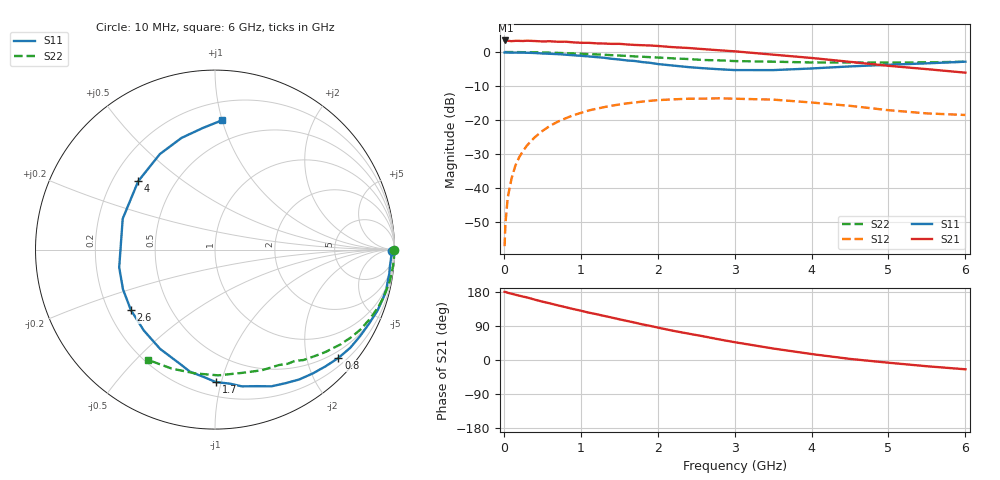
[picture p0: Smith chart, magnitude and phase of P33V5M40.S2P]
! SIEMENS Small Signal Semiconductors
! BFP181
! Si NPN RF Bipolar Junction Transistor in SOT143
! VCE = 3.5 V  IC = 0.4 mA
! Common Emitter S-Parameters:  March  1996
# GHz  S  MA  R  50
!  f  S11  S21  S12  S22
! GHz  MAG  ANG  MAG  ANG  MAG  ANG  MAG  ANG
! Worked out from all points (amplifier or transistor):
!   36 points, 10 MHz to 6 GHz, reference 50 ohm
!   highest |S21| = 3.4 dB at 20 MHz (marker M1)
!   |S21| within 3 dB of that: start of sweep to 2.871 GHz
!   unconditionally stable (mu >= 1): 3.865 GHz to end of sweep
!   at 250 MHz: K = 0.08, MSG = 16.2 dB, |S12| = -29.1 dB
!   at 1.4 GHz: K = 0.42, MSG = 9.1 dB, |S12| = -15.8 dB
!   at 6 GHz: K = 1.48, MAG = 2.1 dB, |S12| = -18.5 dB
!   S11 on the Smith chart (normalised r, x): 10 MHz: open; 800 MHz: 0.35, -2.61; 1.7 GHz: 0.30, -0.96; 2.6 GHz: 0.29, -0.30; 4 GHz: 0.31, +0.35; 6 GHz: 0.33, +1.00
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0.01  0.9837 -0.6  1.453 179.8  0.0014 82.3  0.9994 -0.2
0.02  0.9912 -1.0  1.479 179.8  0.0029 90.8  0.9994 -0.6
0.05  0.9829 -2.2  1.465 177.5  0.0072 91.3  0.998 -1.3
0.1  0.9791 -5.3  1.443 174.9  0.0138 85.6  0.9985 -2.5
0.15  0.9803 -7.9  1.461 172.3  0.0214 83.6  0.9967 -3.8
0.2  0.9784 -10.3  1.459 169.7  0.0285 83.3  0.9966 -5.0
0.3  0.9753 -15.7  1.467 165.2  0.0422 78.8  0.9928 -7.7
0.4  0.9675 -20.4  1.451 159.4  0.0556 75.1  0.9902 -10.1
0.6  0.941 -30.9  1.439 149.4  0.0822 67.4  0.9774 -15.1
0.8  0.9149 -41.3  1.42 139.5  0.1057 60.1  0.9622 -19.9
1.1  0.8625 -57.0  1.366 125.1  0.1379 49.6  0.9332 -26.7
1.5  0.7765 -78.9  1.319 107.5  0.1691 36.6  0.8869 -35.1
1.7  0.7381 -89.6  1.272 98.8  0.1811 30.8  0.8621 -39.0
1.9  0.6938 -101.7  1.248 90.1  0.1916 25.0  0.8407 -42.6
2.2  0.632 -119.0  1.178 77.1  0.2013 17.1  0.8073 -47.8
2.6  0.5769 -144.4  1.102 62.3  0.2062 7.7  0.7632 -54.3
3  0.5429 -169.5  1.024 47.0  0.2058 -1.7  0.7361 -60.8
3.5  0.5422 161.5  0.915 30.4  0.1998 -11.2  0.7212 -68.8
4  0.573 138.3  0.818 15.7  0.1811 -18.6  0.7025 -78.2
4.5  0.6145 120.0  0.717 2.9  0.1618 -24.4  0.7009 -88.5
5.5  0.6817 95.5  0.56 -16.5  0.1252 -22.4  0.7055 -110.0
6  0.7209 87.0  0.497 -24.5  0.1187 -17.6  0.7189 -121.3
